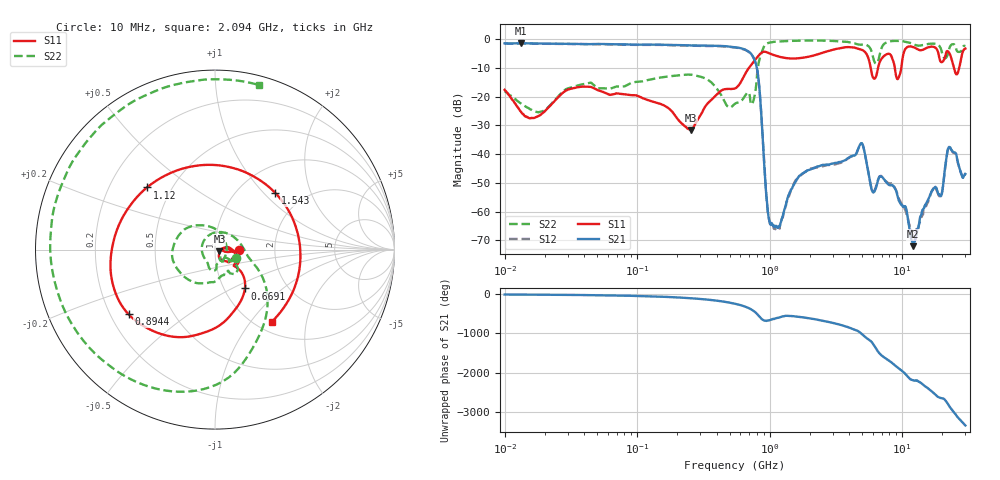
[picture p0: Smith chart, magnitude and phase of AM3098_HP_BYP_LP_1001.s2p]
!Agilent Technologies,E8364B,MY43040894,A.07.50.67
!Agilent E8364B: A.07.50.67
!Date: Wednesday, June 17, 2020 09:20:59
!Correction: S11(Full 2 Port(1,2))
!S21(Full 2 Port(1,2))
!S12(Full 2 Port(1,2))
!S22(Full 2 Port(1,2))
!S2P File: Measurements: S11, S21, S12, S22:Log Frequency Sweep
# Hz S  dB  R 50
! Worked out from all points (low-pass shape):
!   1601 points, 10 MHz to 30 GHz, reference 50 ohm
!   highest |S21| = -1.41 dB at 13.37 MHz (marker M1); lowest = -72.0 dB at 12.13 GHz (marker M2)
!   |S21| within 3 dB of the highest: start of sweep to 698.8 MHz
!   lowest |S11| = -31.6 dB at 254.7 MHz (marker M3), VSWR 1.05, Z = 52.5 - j0.932 ohm
!   |S11| at or under -10 dB: 5.784 GHz to 6.575 GHz (791.4 MHz wide, 12.8 % of centre); 8.804 GHz to 9.851 GHz (1.047 GHz wide, 11.2 % of centre); 24.61 GHz to 26.93 GHz (2.318 GHz wide, 9 % of centre)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
!   |S22| runs from -25.5 to -0.4 dB; largest |S21 - S12| = 0.014
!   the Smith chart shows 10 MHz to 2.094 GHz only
!   S11 on the Smith chart (normalised r, x): 10 MHz: 1.30, -0.01; 669.1 MHz: 1.25, -0.58; 894.4 MHz: 0.27, -0.31; 1.12 GHz: 0.36, +0.34; 1.543 GHz: 1.46, +1.17; 2.094 GHz: 1.17, -1.28
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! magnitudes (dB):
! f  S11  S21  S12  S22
! 10 MHz  -17.6  -1.4  -1.5  -18.1
! 13.37 MHz  -25.4  -1.4  -1.5  -22.5
! 38.04 MHz  -16.6  -1.7  -1.7  -15.8
! 144.7 MHz  -22.3  -1.9  -2.0  -13.4
! 254.7 MHz  -31.6  -2.2  -2.3  -12.4
! 547.7 MHz  -17.1  -2.8  -2.9  -22.5
! 669.1 MHz  -11.3  -3.9  -4.0  -18.9
! 801.2 MHz  -6.4  -10.0  -10.1  -12.9
! 894.4 MHz  -4.4  -37.6  -37.4  -3.1
! 983.6 MHz  -4.8  -62.0  -61.9  -1.3
! 1.12 GHz  -5.8  -64.9  -65.6  -0.9
! 1.543 GHz  -6.7  -50.2  -49.8  -0.6
! 2.084 GHz  -5.8  -45.1  -45.0  -0.5
! 2.094 GHz  -5.8  -45.0  -45.0  -0.5
! 4.903 GHz  -3.6  -36.2  -36.3  -1.9
! 5.989 GHz  -13.1  -53.2  -52.9  -5.7
! 7.926 GHz  -5.1  -50.7  -50.1  -0.9
! 9.302 GHz  -13.8  -55.0  -54.5  -0.6
! 12.13 GHz  -2.7  -72.0  -68.4  -1.7
! 19.61 GHz  -7.9  -54.6  -54.8  -3.4
! 22.56 GHz  -4.6  -37.5  -37.6  -3.7
! 30 GHz  -3.3  -46.9  -46.6  -2.4
